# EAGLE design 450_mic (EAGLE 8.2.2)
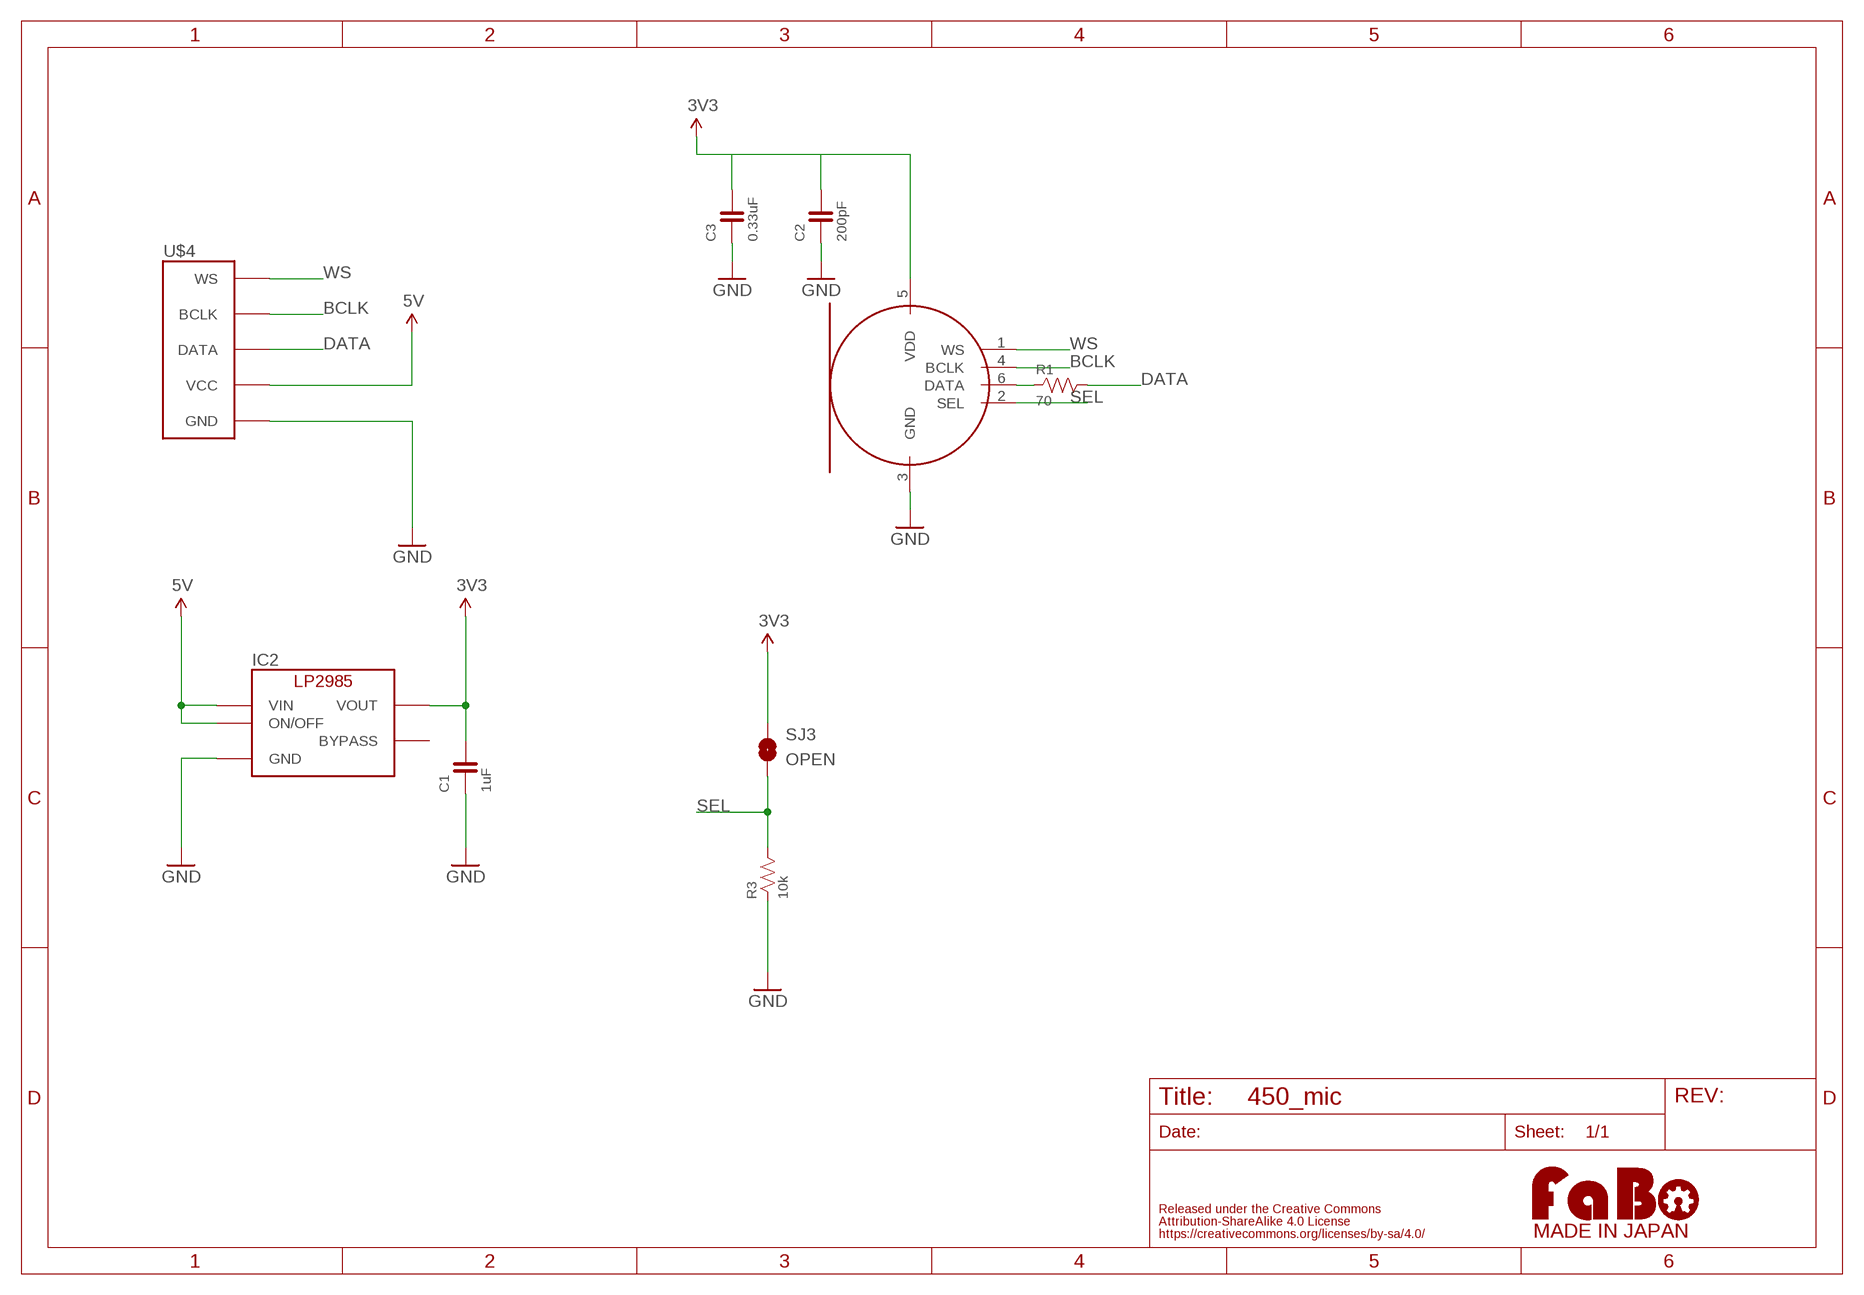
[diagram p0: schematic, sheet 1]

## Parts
C1  1uF  CAPACITOR-0603  [0603]
C2  200pF  CAPACITOR-0603  [0603]
C3  0.33uF  CAPACITOR-0603  [0603]
IC2  LP2985-33DBV  [SOT-23-5]
MIC1  KW-SPH0645  [KNOWLES-SPH0645]
R1  70  RESISTOR-0603  [0603]
R3  10k  RESISTOR-0603  [0603]
SJ3  OPEN  SMD-JUMPER-2-OPEN  [SMD-JUMPER-2-OPEN]
U$3  LOGO_FABO-M_BOTTOM  [LOGO_FABO_MS_BOTTOM]
U$4  FABO_BRICK_I2S  [FABO_BRICK_I2S]

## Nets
3V3: C1.2 C2.2 C3.2 IC2.5(VOUT) MIC1.5(VDD) SJ3.1
5V: IC2.1(VIN) IC2.3(ON/OFF) U$4.VCC
BCLK: MIC1.4(BCLK) U$4.BCLK
DATA: R1.2 U$4.DATA
GND: C1.1 C2.1 C3.1 IC2.2(GND) MIC1.3(GND) R3.1 U$4.GND
N$6: MIC1.6(DATA) R1.1
SEL: MIC1.2(SEL) R3.2 SJ3.2
WS: MIC1.1(WS) U$4.WS
Unconnected: IC2.4(BYPASS)

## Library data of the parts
C1-C3 = FaBo-Capacitor:CAPACITOR: CAPACITOR
IC2 = FaBo-Supply:LP2985: LP2985
MIC1 = FaBo-Mems:KW-SPH0645
R1 R3 = FaBo-Resistors:RESISTOR: RESISTOR
SJ3 = FaBo-Supply:SMD-JUMPER-2
U$3 = FaBo-etc:LOGO_FABO
U$4 = FaBo-Template:FABO_BRICK_I2S

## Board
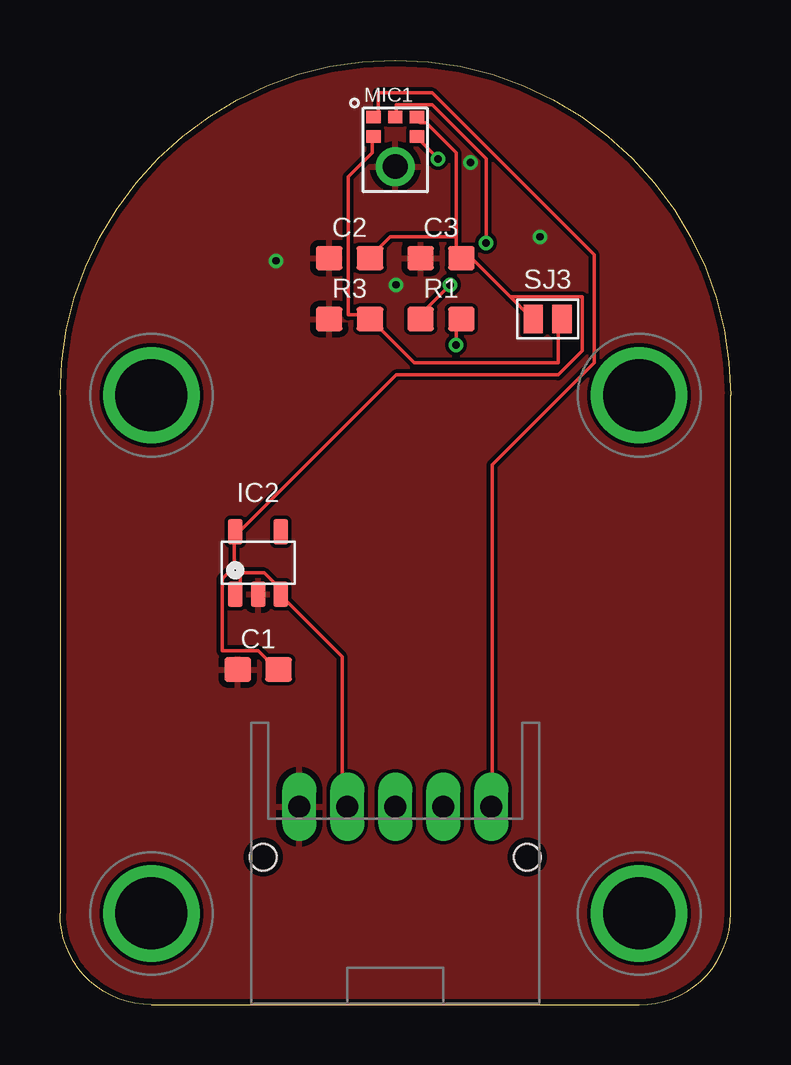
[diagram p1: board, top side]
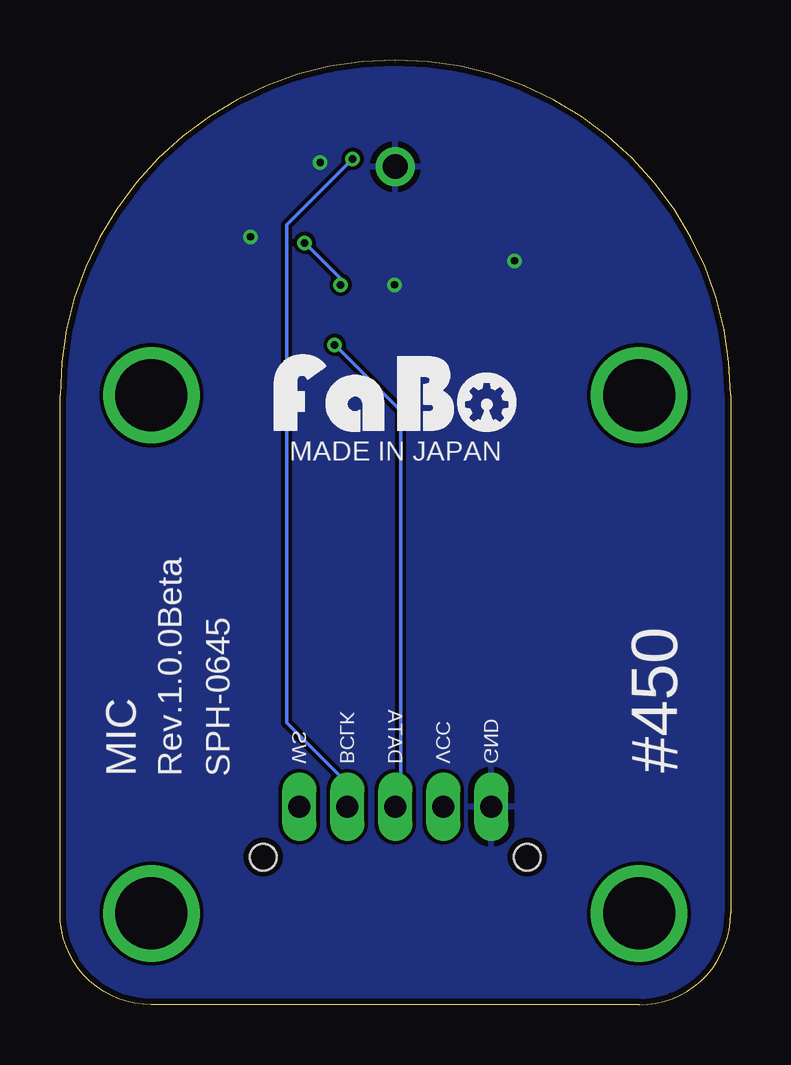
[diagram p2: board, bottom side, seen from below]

Size 27.94 x 39.37 mm. Coordinates in mm from the lower left corner, seen from the top.
Copper layers (1*16): Top 0.035mm / dielectric 1.5mm / Bottom 0.035mm
Design rules "Elecrow_angle": minimum track width 6mil, minimum drill 12mil, track to track 6mil, track to pad 6mil, pad to pad 6mil, via to via 6mil, smd to smd 0mil, copper to edge 10mil, drill to drill 10mil, minimum pad ring 10mil, minimum via ring 6mil, stop-mask expansion 2mil, vias tented up to drill 100mil, thermal gap 10mil

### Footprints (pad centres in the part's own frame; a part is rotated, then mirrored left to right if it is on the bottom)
0603 = smd 1.1 x 1: 1 -0.85,0; 2 0.85,0
SOT-23-5 = smd 0.6 x 1.05: 1 -0.95,-1.3; 2 0,-1.3; 3 0.95,-1.3; 4 0.95,1.3; 5 -0.95,1.3
KNOWLES-SPH0645 = smd 0.6 x 0.522: 1 -0.9,2.074; 2 -0.9,1.252; 4 0.9,1.252; 5 0.9,2.074; 6 0,2.074 | drill 1.024 pad 1.624: 3 0,0
SMD-JUMPER-2-OPEN = smd 0.8 x 1.2: 1 -0.6,0; 2 0.6,0
FABO_BRICK_I2S = drill 0.9 pad 1.422 long: BCLK 2,-9.525; DATA 0,-9.525; GND -4,-9.525; VCC -2,-9.525; WS 4,-9.525 | drill 3 pad 3.81: P$1 -10.16,7.62; P$2 10.16,7.62; P$3 -10.16,-13.97; P$4 10.16,-13.97 | hole 1.1: -5.5,-11.625; 5.5,-11.625

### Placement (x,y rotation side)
C1  8.26,13.97 0 top
C2  12.06,31.11 0 top
C3  15.88,31.11 0 top
IC2  8.26,18.41 0 top
MIC1  13.97,34.92 0 top
R1  15.88,28.57 0 top
R3  12.06,28.57 0 top
SJ3  20.32,28.57 0 top
U$3  13.97,23.5 0 top
U$4  13.97,17.78 0 top

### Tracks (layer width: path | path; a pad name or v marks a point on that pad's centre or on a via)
3V3
  Top 0.152: C1.2 9,14 8.25,14.75 6.75,14.75 6.75,17.75 7.25,18.25 7.25,19.5 IC2.5 7.5,19.75 14,26.25 20.75,26.25 21.75,27.25 21.75,29.5 18.75,29.5 | 16.5,32 16.5,31.25 C3.2 16.75,31 17.25,31 18.75,29.5 | 16.5,32 16.5,35.5 15.25,36.75 15,36.75 MIC1.5 | 16.5,32 13.75,32 13,31.25 C2.2 | 18.75,29.5 19.5,28.75 SJ3.1
5V
  Top 0.152: IC2.1 7.5,17.25 7.5,18 8.5,18 9.25,17.25 IC2.3 9.25,17 11.75,14.5 11.75,8.5 U$4.VCC
BCLK  (via drill 0.3)
  Top 0.152: v15.75,35.25 15,36 MIC1.4
  Bottom 0.152: v15.75,35.25 18.5,32.5 18.5,11.75 16,9.25 16,8.5 U$4.BCLK
DATA  (via drill 0.3)
  Top 0.152: v16.5,27.5 16.5,28.5 R1.2
  Bottom 0.152: v16.5,27.5 13.75,24.75 13.75,8.5 U$4.DATA
GND  (via drill 0.3)
  other vias: 9,31 20,32 14,30 17.1,35.1
  pour Top: 0,0 28,0 28,40 0,40
  pour Bottom: 0,0 28,0 28,40 0,40
N$6  (via drill 0.3)
  Top 0.152: v17.75,31.75 17.75,35.25 15.5,37.5 14,37.5 14,37 MIC1.6 | v16.25,30 15,28.75 R1.1
  Bottom 0.152: v17.75,31.75 16.25,30.25 v16.25,30
SEL
  Top 0.152: MIC1.2 13,36 13,35.5 12,34.5 12,28.75 12.75,28.75 R3.2 13,28.5 14.75,26.75 20.75,26.75 20.75,28.5 SJ3.2
WS
  Top 0.152: MIC1.1 13.25,37 13.25,38 15.5,38 22.25,31.25 22.25,26.75 18,22.5 18,8.5 U$4.WS

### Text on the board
bPlace: MADE IN JAPAN | #450 | SPH-0645 | Rev.1.0.0Beta | MIC

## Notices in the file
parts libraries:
FaBo-etc: Released under the Creative Commons Attribution-ShareAlike 4.0 License
https://creativecommons.org/licenses/by-sa/4.0
FaBo-etc: Released under the Creative Commons
